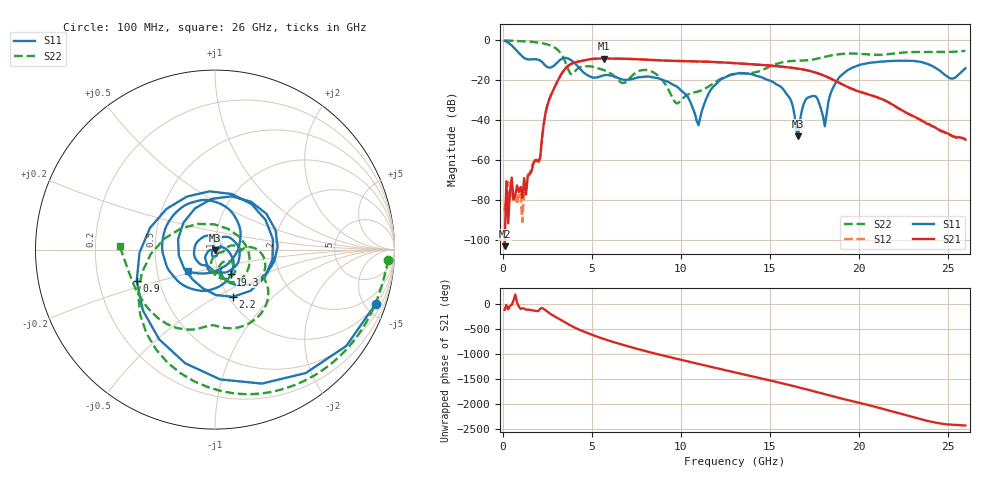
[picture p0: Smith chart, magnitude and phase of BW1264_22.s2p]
!Keysight Technologies,N5245B,MY57181159,A.13.60.06
!Date: Friday, December 18, 2020 23:53:05
!Correction: S11(Full 2 Port(1,2))
!S21(Full 2 Port(1,2))
!S12(Full 2 Port(1,2))
!S22(Full 2 Port(1,2))
!S2P File: Measurements: S11, S21, S12, S22:
# Hz S  dB  R 50
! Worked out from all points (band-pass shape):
!   260 points, 100 MHz to 26 GHz, reference 50 ohm
!   highest |S21| = -9.35 dB at 5.7 GHz (marker M1); lowest = -103.3 dB at 100 MHz (marker M2)
!   |S21| within 3 dB of the highest: 3.782 GHz to 14.27 GHz (10.48 GHz wide, 116 % of centre)
!   lowest |S11| = -48.2 dB at 16.6 GHz (marker M3), VSWR 1.01, Z = 50.1 - j0.372 ohm
!   |S11| at or under -10 dB: 2.009 GHz to 3.225 GHz (1.216 GHz wide, 46.5 % of centre); 3.807 GHz to end of sweep
!   |S22| runs from -31.8 to -0.3 dB; largest |S21 - S12| = 0.00054
!   S11 on the Smith chart (normalised r, x): 100 MHz: 1.04, -5.94; 900 MHz: 0.37, -0.17; 2.2 GHz: 1.05, -0.60; 19.3 GHz: 1.14, -0.32; 26 GHz: 0.72, -0.18
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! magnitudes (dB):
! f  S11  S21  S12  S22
! 100 MHz  -0.5  -103.3  -85.5  -0.3
! 500 MHz  -2.8  -68.9  -73.6  -0.5
! 600 MHz  -3.7  -80.0  -79.6  -0.5
! 900 MHz  -6.6  -76.3  -76.5  -0.6
! 1.3 GHz  -9.5  -77.5  -76.1  -0.8
! 2.2 GHz  -11.0  -49.3  -49.5  -1.6
! 3.1 GHz  -11.0  -20.3  -20.3  -5.2
! 4.5 GHz  -16.0  -10.4  -10.4  -13.3
! 5.7 GHz  -17.7  -9.3  -9.3  -15.2
! 8.8 GHz  -19.4  -10.3  -10.3  -18.6
! 9.8 GHz  -23.5  -10.6  -10.6  -31.8
! 11 GHz  -42.7  -10.8  -10.8  -25.8
! 11.7 GHz  -24.8  -11.0  -11.0  -22.5
! 13.1 GHz  -17.0  -11.7  -11.7  -17.0
! 15.7 GHz  -24.1  -13.5  -13.4  -11.2
! 16.6 GHz  -48.2  -14.4  -14.4  -10.4
! 17.4 GHz  -28.2  -15.9  -15.9  -9.9
! 18.1 GHz  -43.3  -18.1  -18.1  -8.5
! 18.5 GHz  -25.1  -19.7  -19.7  -7.7
! 19.3 GHz  -15.7  -23.3  -23.3  -6.9
! 21.7 GHz  -10.6  -31.3  -31.4  -7.1
! 26 GHz  -14.2  -50.0  -49.6  -5.5
